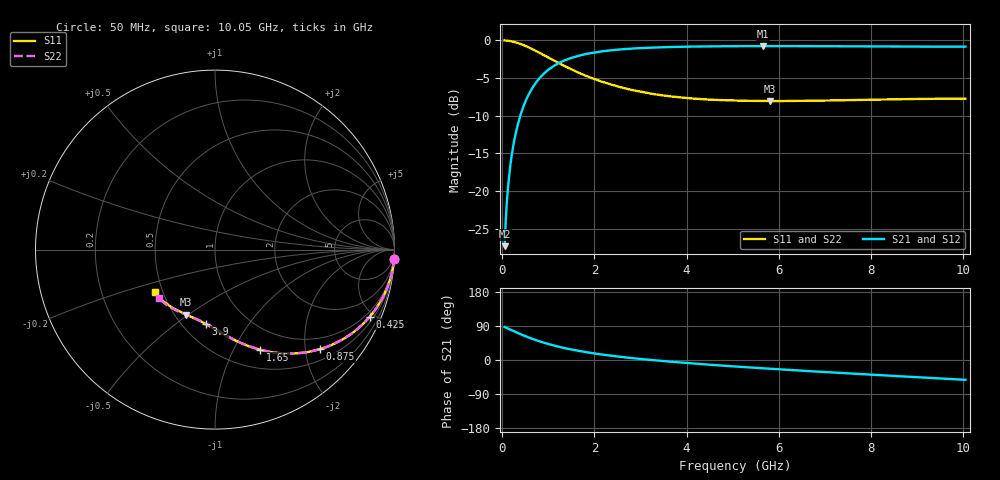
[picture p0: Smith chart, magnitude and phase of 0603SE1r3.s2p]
! AVX Thin Film Operation		Date: August 2001
! Description: Accu-P® Series, Thin Film, SMD, RF Capacitor
! Part Number: 06035J1R3ABT
! 50 MHz  -  10.05 GHz
! Serial Measurements
# mhz S db R 50
!	S11		S21		S12		S22
!	dB	Phase	dB	Phase	dB	Phase	dB	Phase
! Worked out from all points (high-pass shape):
!   401 points, 50 MHz to 10.05 GHz, reference 50 ohm
!   highest |S21| = -0.76 dB at 5.65 GHz (marker M1); lowest = -27.3 dB at 50 MHz (marker M2)
!   |S21| within 3 dB of the highest: 1.032 GHz to end of sweep
!   lowest |S11| = -8.1 dB at 5.8 GHz (marker M3), VSWR 2.31, Z = 28.5 - j24.5 ohm
!   |S11| at or under -10 dB: nowhere
!   |S22| runs from -8.0 to 0.0 dB; largest |S21 - S12| = 0
!   S11 on the Smith chart (normalised r, x): 50 MHz: 1, -40; 425 MHz: 0.74, -4.72; 875 MHz: 0.73, -2.32; 1.65 GHz: 0.72, -1.28; 3.9 GHz: 0.65, -0.65; 10.05 GHz: 0.45, -0.26
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50  -0.01 -2.9  -27.30 87.1  -27.30 87.1  -0.01 -2.9
75  -0.02 -4.3  -23.81 85.7  -23.81 85.7  -0.02 -4.3
125  -0.05 -7.2  -19.44 82.9  -19.44 82.9  -0.05 -7.2
150  -0.07 -8.6  -17.91 81.4  -17.91 81.4  -0.07 -8.6
200  -0.13 -11.4  -15.39 78.6  -15.39 78.6  -0.13 -11.4
300  -0.28 -16.9  -12.08 73.1  -12.08 73.1  -0.28 -16.9
425  -0.54 -23.4  -9.34 66.6  -9.34 66.6  -0.54 -23.4
625  -1.07 -33.0  -6.59 56.9  -6.59 56.9  -1.07 -33.0
875  -1.86 -43.4  -4.58 46.6  -4.58 46.6  -1.86 -43.4
1250  -3.09 -55.7  -2.94 34.2  -2.94 34.2  -3.09 -55.7
1650  -4.26 -65.7  -2.05 24.3  -2.05 24.3  -4.26 -65.6
1725  -4.47 -67.4  -1.93 22.6  -1.93 22.6  -4.46 -67.3
2025  -5.18 -73.2  -1.58 16.9  -1.58 16.9  -5.18 -73.0
2425  -5.98 -79.7  -1.28 10.4  -1.28 10.4  -5.97 -79.4
3400  -7.22 -92.0  -0.92 -1.8  -0.92 -1.8  -7.21 -91.3
3900  -7.59 -97.2  -0.84 -6.9  -0.84 -6.9  -7.58 -96.3
5050  -7.99 -107.6  -0.77 -17.1  -0.77 -17.1  -7.97 -106.0
5650  -8.04 -112.5  -0.76 -21.9  -0.76 -21.9  -8.03 -110.5
5800  -8.05 -114.0  -0.76 -23.0  -0.76 -23.0  -8.03 -112.0
6725  -8.01 -120.9  -0.77 -29.8  -0.77 -29.8  -7.99 -118.4
8400  -7.83 -133.2  -0.81 -41.4  -0.81 -41.4  -7.80 -129.2
10050  -7.72 -144.8  -0.84 -52.3  -0.84 -52.3  -7.68 -139.4
